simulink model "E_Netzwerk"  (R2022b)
settings: Solver=ode45  StartTime=0.0  StopTime=0.15  MaxStep=1e-4  MinStep=1e-5  RelTol=1e-4
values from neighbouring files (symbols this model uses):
  dr = -10    [Esys_Parameter.m]
  te = .05    (= 0.05)    [Esys_Parameter.m]
  ts1 = 0.03    [Esys_Parameter.m]
  ts2 = 0.11    [Esys_Parameter.m]
  UeR = 5    [Esys_Parameter.m]
  Us = 4    [Esys_Parameter.m]
  Usinus = 1    [Esys_Parameter.m]
  UsR = 5    [Esys_Parameter.m]
  we = 1000    [Esys_Parameter.m]
undefined symbols (not defined in the file or in its folder): Asys, bdsys, busys, k, par, R_PI, R_PID, UaR
libraries: cstblocks x4, simulink x2

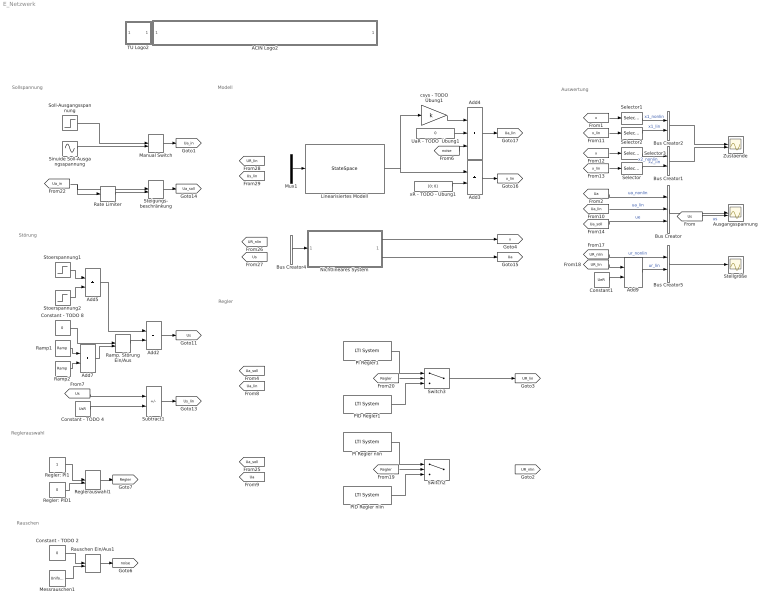
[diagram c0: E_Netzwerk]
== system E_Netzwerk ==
  note: Reglerauswahl
  note: Rauschen
  note: Störung
  note: Sollspannung
  note: Auswertung
  note: Modell
  note: Regler
  ACIN Logo2 : Subsystem
      mask init:
      | s = get_param(gcb,'UserData');
  Add{2..3,5,7,9} (5 alike) : Sum
  Add4 : Sum  Inputs=+++
  Ausgangsspannung : Scope  NumInputPorts=2
  Bus Creator : BusCreator  Inputs=3
  Bus Creator{1..2,4..5} (4 alike) : BusCreator  Inputs=2
  Constant - TODO 2 : Constant  Value=0
  Constant - TODO 4 : Constant  Value=UsR
  Constant - TODO 8 : Constant  Value=0
  Constant1 : Constant  Value=UeR
  Linearisiertes Modell : StateSpace  A=Asys  B=[busys bdsys]  C=eye(2)  D=zeros(2)  InitialCondition=[0;0]
  Manual Switch : ManualSwitch
  Messrauschen1 : UniformRandomNumber  Minimum=-5e-2  Maximum=5e-2
  Mux1 : Mux  Inputs=2
  Nichtlineares System : Subsystem
  PI Regler nlin : cstblocks/LTI System  sys=tf(R_PI.num{1},R_PI.den{1})  IC=[]
  PI Regler1 : cstblocks/LTI System  sys=tf(R_PI.num{1},R_PI.den{1})  IC=[]
  PID Regler nlin : cstblocks/LTI System  sys=tf(R_PID.num{1},R_PID.den{1})  IC=[]
  PID Regler1 : cstblocks/LTI System  sys=tf(R_PID.num{1},R_PID.den{1})  IC=[]
  Ramp. Störung Ein/Aus : ManualSwitch
  Ramp1 : simulink/Sources/Ramp  slope=dr  start=tsr1  InitialOutput=0
  Ramp2 : simulink/Sources/Ramp  slope=-dr  start=tsr2  InitialOutput=0
  Rate Limiter : RateLimiter  RisingSlewLimit=200  FallingSlewLimit=-200  SampleTimeMode=inherited
  Rauschen Ein/Aus1 : ManualSwitch  CurrentSetting=0
  Regler: PI1 : Constant
  Regler: PID1 : Constant  Value=0
  Reglerauswahl1 : ManualSwitch
  Selector : Selector  InputPortWidth=2  IndexOptions=Index vector (dialog)  Indices=2  OutputSizes=1
  Selector1 : Selector  InputPortWidth=2  IndexOptions=Index vector (dialog)  Indices=1  OutputSizes=1
  Selector2 : Selector  InputPortWidth=2  IndexOptions=Index vector (dialog)  Indices=1  OutputSizes=1
  Selector3 : Selector  InputPortWidth=2  IndexOptions=Index vector (dialog)  Indices=2  OutputSizes=1
  Sinuide Soll-Ausgangsspannung : Sin  Amplitude=Usinus  Bias=UaR  Frequency=we  SampleTime=0
  Soll-Ausgangsspannung : Step  Time=te  Before=UaR  After=UaR+2  SampleTime=0
  Steigungs- beschränkung : ManualSwitch
  Stellgröße : Scope
  Stoerspannung1 : Step  Time=ts1  Before=UsR  After=Us  SampleTime=0
  Stoerspannung2 : Step  Time=ts2  After=UsR-Us  SampleTime=0
  Subtract1 : Sum  Inputs=+-
  Switch2 : Switch  Criteria=u2 ~= 0
  Switch3 : Switch  Criteria=u2 ~= 0
  TU Logo2 : Subsystem
      mask init:
      | s = get_param(gcb,'UserData');
  UaR - TODO  Übung1 : Constant  Value=0
  Zustaende : Scope  NumInputPorts=2
  csys - TODO Übung1 : Gain  Gain=k  Multiplication=Matrix(K*u)
  xR - TODO - Übung1 : Constant  Value=[0; 0]
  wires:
  Regler: PID1/1 -> Reglerauswahl1/2
  Reglerauswahl1/1 -> [Regler]
  Messrauschen1/1 -> Rauschen Ein/Aus1/2
  Constant - TODO 2/1 -> Rauschen Ein/Aus1/1
  Regler: PI1/1 -> Reglerauswahl1/1
  Rauschen Ein/Aus1/1 -> [noise]
  Add7/1 -> Ramp. Störung Ein/Aus/2
  Ramp1/1 -> Add7/1
  Ramp. Störung Ein/Aus/1 -> Add2/2
  Ramp2/1 -> Add7/2
  Add5/1 -> Add2/1
  [Us] -> Subtract1/1
  Stoerspannung2/1 -> Add5/2
  Stoerspannung1/1 -> Add5/1
  Constant - TODO 4/1 -> Subtract1/2
  Constant - TODO 8/1 -> Ramp. Störung Ein/Aus/1
  Add2/1 -> [Us]
  Subtract1/1 -> [Us_lin]
  Soll-Ausgangsspannung/1 -> Manual Switch/1
  Rate Limiter/1 -> Steigungs- beschränkung/2
  Manual Switch/1 -> [Ua_in]
  Sinuide Soll-Ausgangsspannung/1 -> Manual Switch/2
  [Ua_in] -> Rate Limiter/1, Steigungs- beschränkung/1
  Steigungs- beschränkung/1 -> [Ua_soll]
  [x_lin] -> Selector/1
  Selector2/1 -> Bus Creator2/2  "x1_lin"
  [Ua_soll] -> Bus Creator/3  "ue"
  Constant1/1 -> Add9/2
  Add9/1 -> Bus Creator5/2  "ur_lin"
  Bus Creator5/1 -> Stellgröße/1
  [Ua_lin] -> Bus Creator/2  "ua_lin"
  [Us] -> Ausgangsspannung/2  "us"
  Bus Creator/1 -> Ausgangsspannung/1
  Selector/1 -> Bus Creator1/2  "x2_lin"
  [UR_lin] -> Add9/1
  [UR_nlin] -> Bus Creator5/1  "ur_nonlin"
  Bus Creator1/1 -> Zustaende/2
  [x_lin] -> Selector2/1
  Selector3/1 -> Bus Creator1/1  "x2_nonlin"
  Selector1/1 -> Bus Creator2/1  "x1_nonlin"
  [x] -> Selector1/1
  Bus Creator2/1 -> Zustaende/1
  [x] -> Selector3/1
  [Ua] -> Bus Creator/1  "ua_nonlin"
  [noise] -> Add4/3
  UaR - TODO  Übung1/1 -> Add4/2
  Add3/1 -> [x_lin]
  csys - TODO Übung1/1 -> Add4/1
  Add4/1 -> [Ua_lin]
  Linearisiertes Modell/1 -> csys - TODO Übung1/1, Add3/1
  Mux1/1 -> Linearisiertes Modell/1
  xR - TODO - Übung1/1 -> Add3/2
  PID Regler nlin/1 -> Switch2/3
  ? -> PI Regler nlin/1, PID Regler nlin/1
  PI Regler1/1 -> Switch3/1
  [Regler] -> Switch2/2
  PI Regler nlin/1 -> Switch2/1
  PID Regler1/1 -> Switch3/3
  Switch3/1 -> [UR_lin]
  [Regler] -> Switch3/2
  ? -> PI Regler1/1, PID Regler1/1
  Bus Creator4/1 -> Nichtlineares System/1(u)
  Nichtlineares System/1(x) -> [x]
  Nichtlineares System/2(Ua) -> [Ua]

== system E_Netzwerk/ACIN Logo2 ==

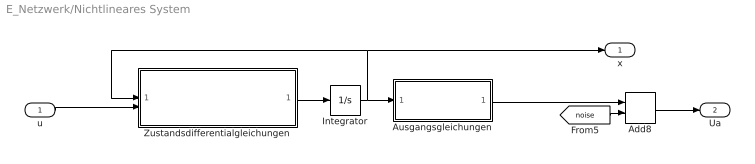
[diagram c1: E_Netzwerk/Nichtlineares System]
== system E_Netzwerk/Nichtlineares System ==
  u : Inport
  Add8 : Sum
  Ausgangsgleichungen : MATLAB Function  TreatAsAtomicUnit=on
  Integrator : Integrator  InitialCondition=par.x0
  Zustandsdifferentialgleichungen : MATLAB Function  TreatAsAtomicUnit=on
  x : Outport
  Ua : Outport  Port=2
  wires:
  Integrator/1 -> x/1, Zustandsdifferentialgleichungen/1(x), Ausgangsgleichungen/1(x)
  Zustandsdifferentialgleichungen/1(dx) -> Integrator/1
  Ausgangsgleichungen/1(y) -> Add8/1
  [noise] -> Add8/2
  u/1 -> Zustandsdifferentialgleichungen/2(u)
  Add8/1 -> Ua/1

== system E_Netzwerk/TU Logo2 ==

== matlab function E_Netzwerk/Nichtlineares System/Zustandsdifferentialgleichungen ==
function dx = Esys_f(x,u,par)
%#codegen
coder.allowpcode('plain');
    dx = Esys_f_mfun(x,u,par);
return;

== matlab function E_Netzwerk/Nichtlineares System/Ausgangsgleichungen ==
function y = Esys_h(x,par)
%#codegen
coder.allowpcode('plain');
    y = Esys_h_mfun(x,par);
return;
